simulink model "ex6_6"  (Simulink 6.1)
settings: Solver=ode15s  SolverMode=SingleTasking  StartTime=0.0  StopTime=1000  RelTol=1e-3  AbsTol=1e-6
undefined symbols (not defined in the file or in its folder): DiscIntNeverNeededParam
libraries: simulink x1

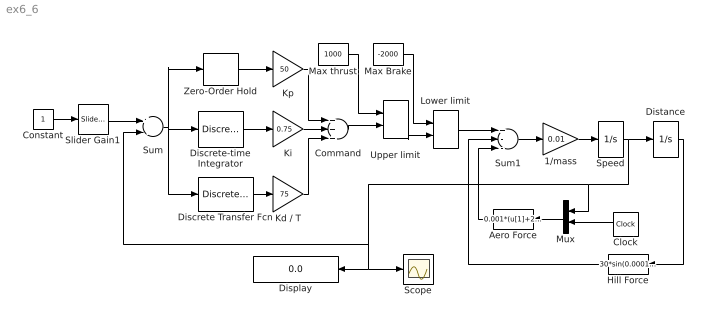
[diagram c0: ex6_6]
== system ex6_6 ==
  1/mass : Gain  Gain=0.01
  Aero Force : Fcn  Orientation=left  Expr=0.001*(u[1]+20*sin(0.01*u[2]))^2
  Clock : Clock
  Command : Sum  Inputs=+++
  Constant : Constant
  Discrete Transfer Fcn : DiscreteTransferFcn  Numerator=[1 -1]  Denominator=[1 0]  SampleTime=0.5
  Discrete-time Integrator : DiscreteIntegrator  SampleTime=0.5  LimitOutput=on  UpperSaturationLimit=100  LowerSaturationLimit=-100  ICPrevOutput=DiscIntNeverNeededParam  ICPrevScaledInput=DiscIntNeverNeededParam
  Display : Display
  Distance : Integrator
  Hill Force : Fcn  Orientation=left  Expr=30*sin(0.0001*u[1])
  Kd / T : Gain  Gain=75
  Ki : Gain  Gain=0.75
  Kp : Gain  Gain=50
  Lower limit : MinMax  Function=max  Inputs=2
  Max Brake : Constant  Value=-2000
  Max thrust : Constant  Value=1000
  Mux : Mux  Orientation=left  Inputs=2
  Scope : Scope
  Slider Gain1 : simulink/Math Operations/Slider Gain  low=0  gain=80  high=100
  Speed : Integrator
  Sum : Sum  Inputs=+-
  Sum1 : Sum  Inputs=+--
  Upper limit : MinMax  Inputs=2
  Zero-Order Hold : ZeroOrderHold  SampleTime=0.5
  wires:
  Speed/1 -> Distance/1, Scope/1, Display/1, Sum/2, Mux/1
  Clock/1 -> Mux/2
  Lower limit/1 -> Sum1/1
  Max Brake/1 -> Lower limit/1
  Max thrust/1 -> Upper limit/1
  Upper limit/1 -> Lower limit/2
  1/mass/1 -> Speed/1
  Sum1/1 -> 1/mass/1
  Distance/1 -> Hill Force/1
  Hill Force/1 -> Sum1/2
  Aero Force/1 -> Sum1/3
  Mux/1 -> Aero Force/1
  Zero-Order Hold/1 -> Kp/1
  Discrete-time Integrator/1 -> Ki/1
  Sum/1 -> Discrete-time Integrator/1, Zero-Order Hold/1, Discrete Transfer Fcn/1
  Discrete Transfer Fcn/1 -> Kd / T/1
  Kp/1 -> Command/1
  Ki/1 -> Command/2
  Kd / T/1 -> Command/3
  Command/1 -> Upper limit/2
  Constant/1 -> Slider Gain1/1
  Slider Gain1/1 -> Sum/1
